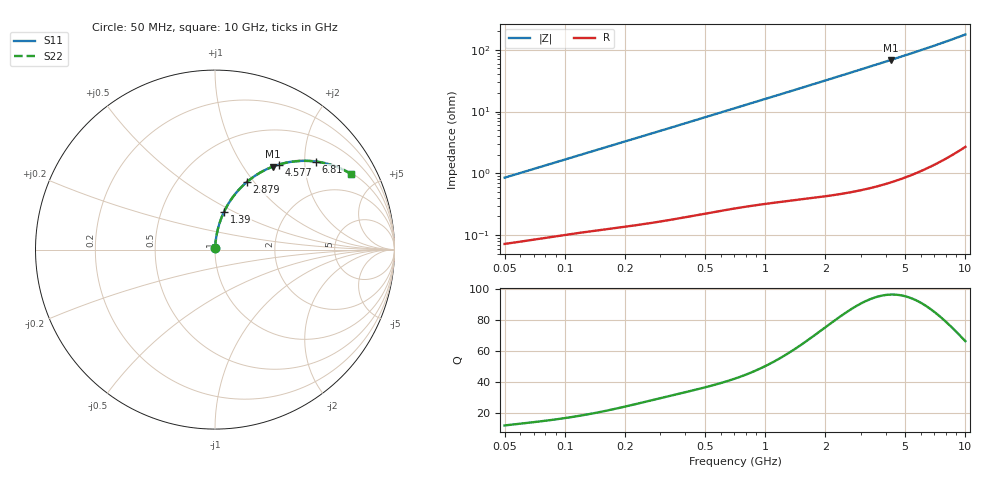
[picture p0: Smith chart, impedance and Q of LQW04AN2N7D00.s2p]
!Murata Part Number: LQW04AN2N7D00
!These Parameters are Measured in Series Mode Connection
!  o--[Z]--o
!Port1  Port2
!  o-------o
!Freq. Start=50[MHz] Stop=10[GHz], 401[Steps]
# Hz S RI R 50
!Freq.(Hz)	S 11(Real)	S 11(Imag)	S 21(Real)	S 21(Imag)	S 12(Real)	S 12(Imag)	S 22(Real)	S 22(Imag)
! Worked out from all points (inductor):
!   401 points, 50 MHz to 10 GHz, reference 50 ohm
!   read as one part in series: L = 2.67 nH near 51.34 MHz
!   highest Q = 96.6 at 4.227 GHz (marker M1), where L = 2.57 nH
!   S11 on the Smith chart (normalised r, x): 50 MHz: 1.00, +0.02; 1.39 GHz: 1.01, +0.44; 2.879 GHz: 1.01, +0.92; 4.577 GHz: 1.02, +1.49; 6.81 GHz: 1.03, +2.27; 10 GHz: 1.05, +3.56
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5e7  0.000786 0.00844  0.9992 -0.00844  0.9992 -0.00844  0.000786 0.00844
5.134228e7  0.000798 0.00866  0.9992 -0.00866  0.9992 -0.00866  0.000798 0.00866
1.214486e8  0.00149 0.02  0.9985 -0.02  0.9985 -0.02  0.00149 0.02
1.956524e8  0.00236 0.0319  0.9976 -0.0319  0.9976 -0.0319  0.00236 0.0319
2.949953e8  0.00391 0.0476  0.9961 -0.0476  0.9961 -0.0476  0.00391 0.0476
4.689809e8  0.00778 0.0749  0.9922 -0.0749  0.9922 -0.0749  0.00778 0.0749
7.071068e8  0.0153 0.1114  0.9847 -0.1114  0.9847 -0.1114  0.0153 0.1114
9.978194e8  0.0278 0.1546  0.9722 -0.1546  0.9722 -0.1546  0.0278 0.1546
1.389525e9  0.05 0.2099  0.95 -0.2099  0.95 -0.2099  0.05 0.2099
1.717543e9  0.073 0.253  0.927 -0.253  0.927 -0.253  0.073 0.253
2.23851e9  0.1164 0.3145  0.8836 -0.3145  0.8836 -0.3145  0.1164 0.3145
2.879108e9  0.1781 0.377  0.8219 -0.377  0.8219 -0.377  0.1781 0.377
3.465724e9  0.2392 0.4214  0.7608 -0.4214  0.7608 -0.4214  0.2392 0.4214
4.171863e9  0.3145 0.4592  0.6855 -0.4592  0.6855 -0.4592  0.3145 0.4592
4.22749e9  0.3204 0.4615  0.6796 -0.4615  0.6796 -0.4615  0.3204 0.4615
4.577181e9  0.357 0.474  0.643 -0.474  0.643 -0.474  0.357 0.474
5.583245e9  0.4569 0.4928  0.5431 -0.4928  0.5431 -0.4928  0.4569 0.4928
6.207365e9  0.5133 0.4943  0.4867 -0.4943  0.4867 -0.4943  0.5133 0.4943
6.810442e9  0.5632 0.4902  0.4368 -0.4902  0.4368 -0.4902  0.5632 0.4902
8.090191e9  0.6541 0.4693  0.3459 -0.4693  0.3459 -0.4693  0.6541 0.4693
9.48396e9  0.7323 0.4356  0.2677 -0.4356  0.2677 -0.4356  0.7323 0.4356
1e10  0.7565 0.4217  0.2435 -0.4217  0.2435 -0.4217  0.7565 0.4217
